(* Logix 5000 DataType export Get_Member; software revision 32.01 *)

TYPE Get_Member :
STRUCT
   Address : SINT;   // 1-31 = Address 1A-31A, 32-62 = Address 1B-31B
   Null : SINT;
END_STRUCT
END_TYPE
